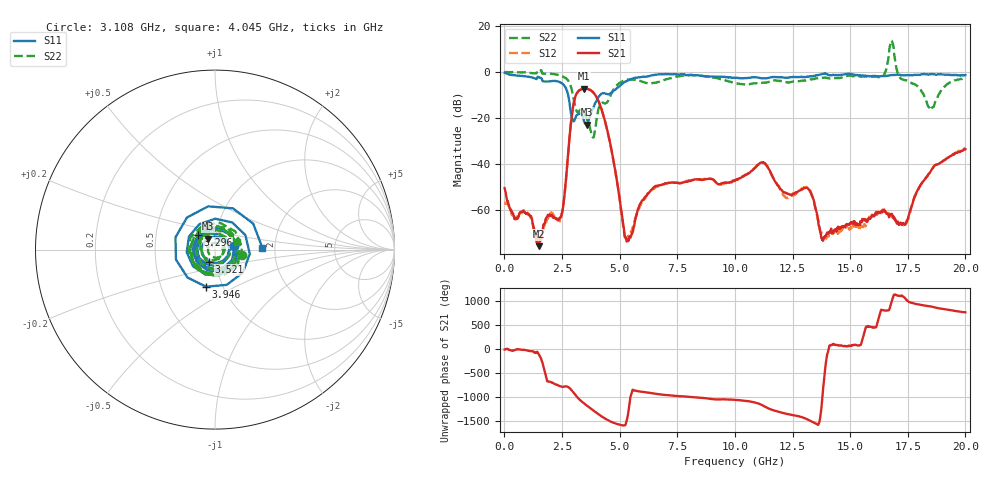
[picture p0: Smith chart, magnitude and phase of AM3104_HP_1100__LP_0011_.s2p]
!Created with skrf (http://scikit-rf.org).
# Hz S RI R 50.0
!freq ReS11 ImS11 ReS21 ImS21 ReS12 ImS12 ReS22 ImS22
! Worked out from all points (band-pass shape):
!   1601 points, 10 MHz to 20 GHz, reference 50 ohm
!   highest |S21| = -7.20 dB at 3.458 GHz (marker M1); lowest = -75.5 dB at 1.484 GHz (marker M2)
!   |S21| within 3 dB of the highest: 3.097 GHz to 3.955 GHz (857.2 MHz wide, 24.3 % of centre)
!   lowest |S11| = -22.8 dB at 3.571 GHz (marker M3), VSWR 1.16, Z = 45.8 + j5.56 ohm
!   |S11| at or under -10 dB: 2.765 GHz to 4.154 GHz (1.389 GHz wide, 40.1 % of centre)
!   |S22| runs from -28.5 to 13.6 dB; largest |S21 - S12| = 0.015
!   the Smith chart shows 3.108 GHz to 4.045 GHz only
!   S11 on the Smith chart (normalised r, x): 3.108 GHz: 1.24, +0.04; 3.296 GHz: 0.81, +0.13; 3.521 GHz: 0.93, -0.13; 3.946 GHz: 0.83, -0.36; 4.045 GHz: 1.72, +0.03
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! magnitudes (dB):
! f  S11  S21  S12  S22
! 10 MHz  -0.4  -50.3  -56.6  -0.1
! 1.484 GHz  -2.2  -75.5  -73.4  0.8
! 2.471 GHz  -4.8  -62.5  -62.5  -1.8
! 3.108 GHz  -19.2  -9.9  -9.9  -16.4
! 3.296 GHz  -18.0  -7.7  -7.8  -16.4
! 3.346 GHz  -18.6  -7.5  -7.5  -16.4
! 3.458 GHz  -21.4  -7.2  -7.2  -18.0
! 3.521 GHz  -22.5  -7.2  -7.3  -19.3
! 3.571 GHz  -22.8  -7.2  -7.3  -20.4
! 3.946 GHz  -13.5  -10.1  -10.1  -24.4
! 4.045 GHz  -11.5  -11.9  -11.9  -17.9
! 5.307 GHz  -3.9  -73.5  -71.4  -3.3
! 6.682 GHz  -1.1  -49.2  -49.4  -4.4
! 10.01 GHz  -2.6  -47.1  -46.8  -4.8
! 11.2 GHz  -2.8  -39.1  -39.4  -4.7
! 13.34 GHz  -2.0  -53.7  -53.2  -3.3
! 13.83 GHz  -0.9  -73.2  -70.5  -2.6
! 16.35 GHz  -1.8  -60.3  -61.1  -2.3
! 16.68 GHz  -1.5  -62.7  -61.5  7.1
! 17.4 GHz  -1.4  -66.1  -65.7  -3.6
! 18.48 GHz  -0.9  -43.4  -43.5  -16.4
! 20 GHz  -1.4  -33.5  -33.1  -2.7
